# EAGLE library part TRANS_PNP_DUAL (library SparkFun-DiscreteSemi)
Dual PNP Transistors in Single Package The BCM857BS puts two PNP transistors in a single package. Bipolar (BJT) Transistor Array 2 PNP (Dual) 45V 100mA 100MHz 200mW Surface Mount SOT-363 Datasheet SparkFun Products: SparkFun Pi Servo HAT V2
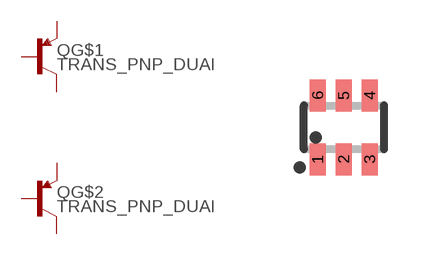
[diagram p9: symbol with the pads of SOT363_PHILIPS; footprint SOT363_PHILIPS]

Designator prefix Q; gates G$1=PNP G$2=PNP

## TRANS_PNP_DUALSOT-363 (PROD_ID: TRANS-14386)  [SOT363_PHILIPS]
1  G$1:E  pas
2  G$1:B  pas
3  G$2:C  pas
4  G$2:E  pas
5  G$2:B  pas
6  G$1:C  pas

## Footprint SOT363_PHILIPS (pad centres in mm)
Small Outline Transistor; 6 leads Philips Semiconductors, SOT363.pdf
smd 0.4 x 0.8: 1 -0.65,-0.8; 2 0,-0.8; 3 0.65,-0.8; 4 0.65,0.8; 5 0,0.8; 6 -0.65,0.8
